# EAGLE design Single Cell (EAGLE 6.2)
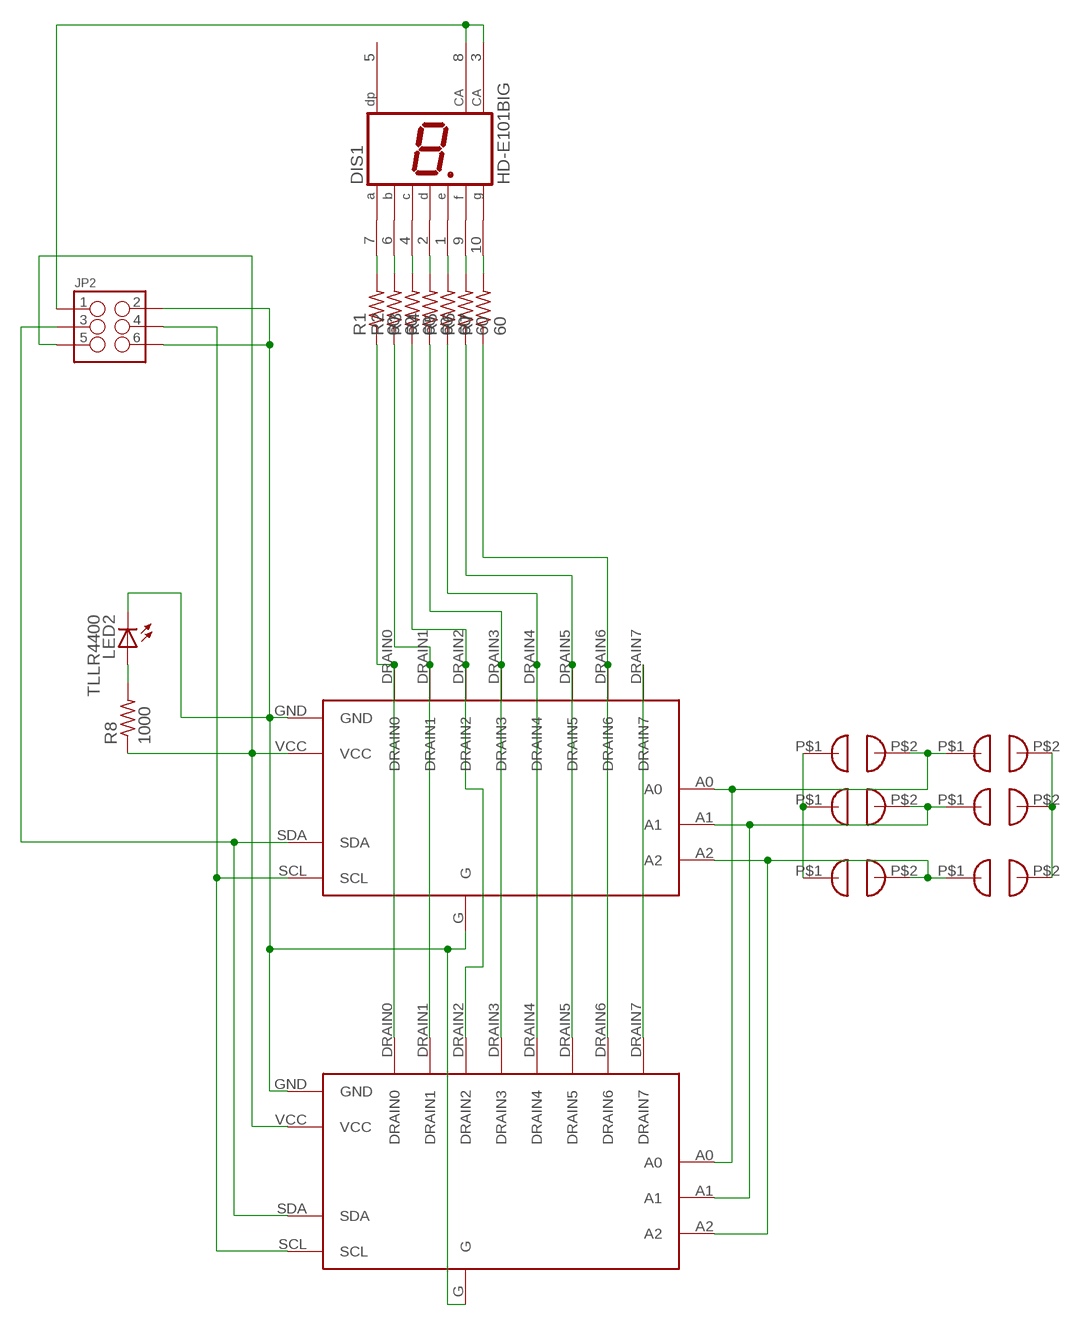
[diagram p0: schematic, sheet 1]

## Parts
DIS1  HD-E101BIG  HD-E101BACKWARDS  [7SEGMENT_BACKWARDS]
JP2  M03X2SHROUD  [2X3-SHROUDED]
LED2  TLLR4400  [LED3MM]
R1  60  R-US_0207/15  [0207/15]
R2  60  R-US_0207/15  [0207/15]
R3  60  R-US_0207/15  [0207/15]
R4  60  R-US_0207/15  [0207/15]
R5  60  R-US_0207/15  [0207/15]
R6  60  R-US_0207/15  [0207/15]
R7  60  R-US_0207/15  [0207/15]
R8  1000  R-US_0207/15  [0207/15]
U$1  SOLDER_JUMPER  [SOLDER_JUMPER]
U$2  LED_DRIVERBOARDADAFRUIT  [DRIVER_BOARD_ADAFRUIT]
U$3  SOLDER_JUMPER  [SOLDER_JUMPER]
U$4  SOLDER_JUMPER  [SOLDER_JUMPER]
U$5  SOLDER_JUMPER  [SOLDER_JUMPER]
U$6  SOLDER_JUMPER  [SOLDER_JUMPER]
U$7  SOLDER_JUMPER  [SOLDER_JUMPER]
U$8  LED_DRIVERBOARD  [DRIVER_BOARD]

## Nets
GND: JP2.2 JP2.6 LED2.K(C) U$1.P$1 U$2.G U$2.GND U$4.P$1 U$6.P$1 U$8.G U$8.GND
N$1: DIS1.7(A) R1.2
N$2: DIS1.6(B) R2.2
N$3: DIS1.4(C) R3.2
N$4: DIS1.2(D) R4.2
N$5: DIS1.1(E) R5.2
N$6: DIS1.9(F) R6.2
N$7: DIS1.10(G) R7.2
N$8: R1.1 U$2.DRAIN0 U$8.DRAIN0
N$9: R2.1 U$2.DRAIN1 U$8.DRAIN1
N$10: R3.1 U$2.DRAIN2 U$8.DRAIN2
N$11: R4.1 U$2.DRAIN3 U$8.DRAIN3
N$12: R5.1 U$2.DRAIN4 U$8.DRAIN4
N$13: R6.1 U$2.DRAIN5 U$8.DRAIN5
N$14: R7.1 U$2.DRAIN6 U$8.DRAIN6
N$15: U$2.A1 U$4.P$2 U$5.P$1 U$8.A1
N$16: U$2.A2 U$6.P$2 U$7.P$1 U$8.A2
N$17: U$2.DRAIN7 U$8.DRAIN7
N$18: LED2.A R8.2
N$29: U$1.P$2 U$2.A0 U$3.P$1 U$8.A0
SDA: JP2.3 U$2.SDA U$8.SDA
SSCL: JP2.4 U$2.SCL U$8.SCL
VCC5: JP2.5 R8.1 U$2.VCC U$3.P$2 U$5.P$2 U$7.P$2 U$8.VCC
VCC12: DIS1.3(CA) DIS1.8(CA) JP2.1
Unconnected: DIS1.5(DP)

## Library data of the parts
DIS1 = Parts:HD-E101: LED DISPLAY 1-character 7 segment, decimal point right
JP2 = Ben-SF-Con:M03X2: 2x3 .1" header. Shrouded, with keying- CONN-10681 SMT- CONN-11415 Pogo pins- HW-11044; PROD_ID: CONN-10681
LED2 = led:TLLR4400: Low Current (2mA) LED 3 mm Tinted Diffused Package color RED; MF: VISHAY SEMICONDUCTOR; OC_FARNELL: 1612437
R1-R8 = Ben-rcl:R-US_: RESISTOR, American symbol
U$1 U$3-U$7 = Parts:SOLDER_JUMPER
U$2 U$8 = Parts:LED_DRIVERBOARD

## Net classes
0 default: width 0.001 mm

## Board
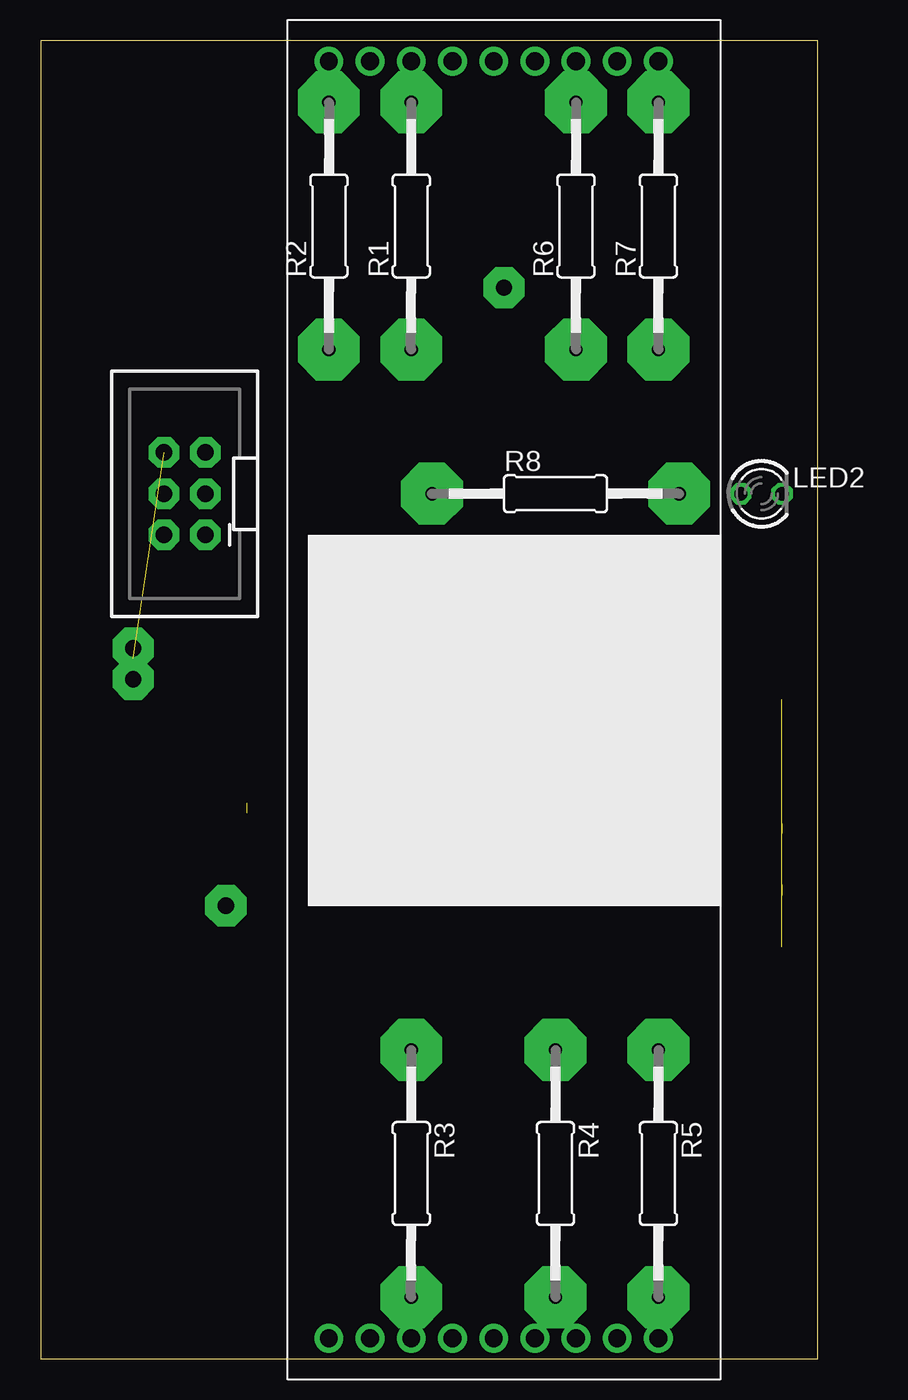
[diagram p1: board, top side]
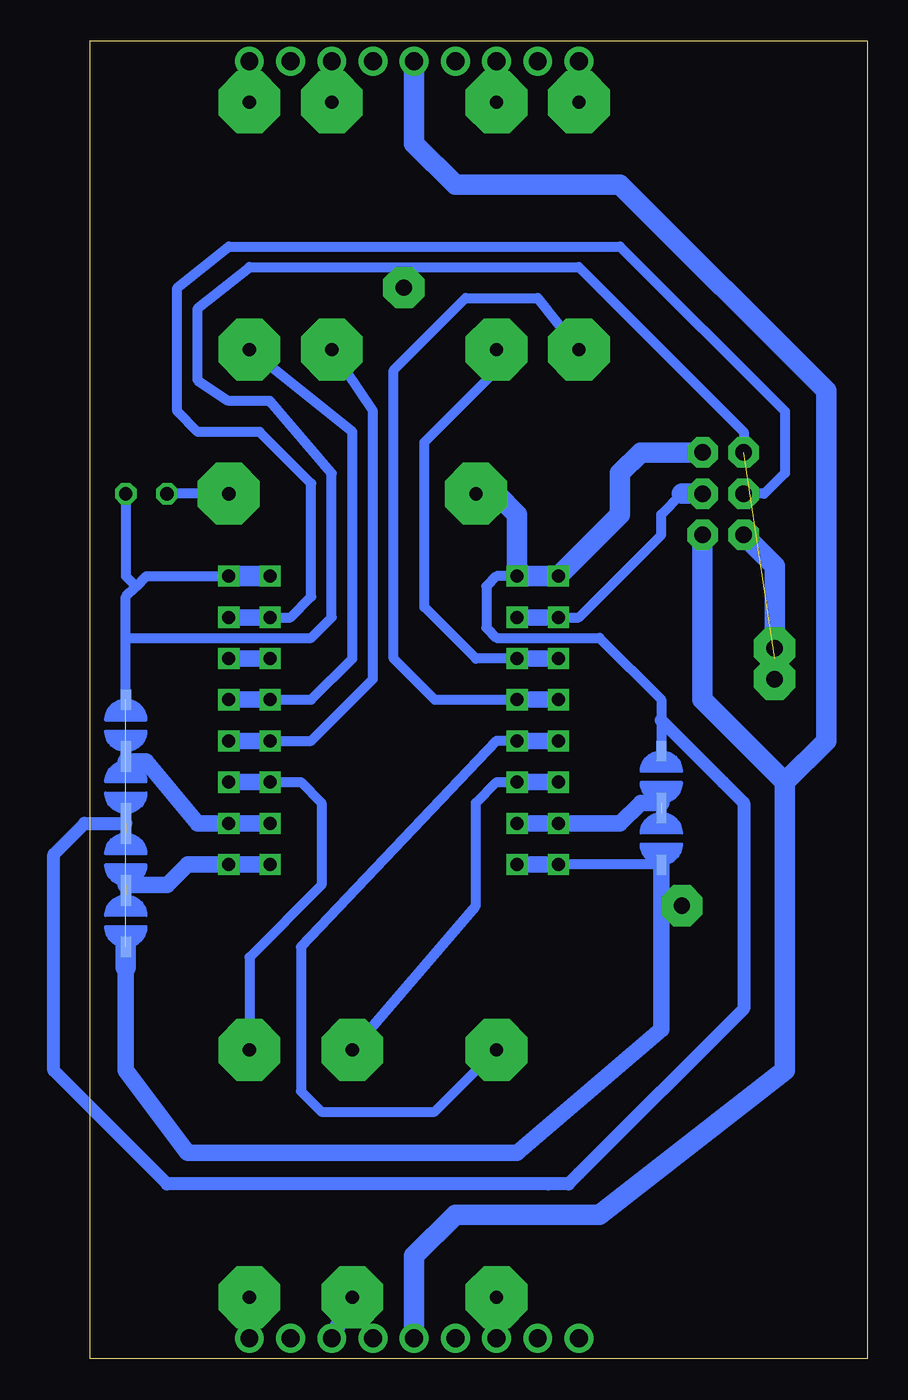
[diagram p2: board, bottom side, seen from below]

Size 47.93 x 81.27 mm. Coordinates in mm from the lower left corner, seen from the top.
Outline: 0,0 47.93,0 47.93,81.27 0,81.27 0,0
Copper layers (1*16): Top 0.035mm / dielectric 1.5mm / Bottom 0.035mm
Design rules: minimum track width 10mil, minimum drill 24mil, track to track 10mil, track to pad 10mil, pad to pad 10mil, via to via 10mil, smd to smd 10mil, copper to edge 40mil, drill to drill 8mil, minimum pad ring 10mil, minimum via ring 8mil, stop-mask expansion 4mil, vias tented up to drill 0mil, thermal gap 10mil

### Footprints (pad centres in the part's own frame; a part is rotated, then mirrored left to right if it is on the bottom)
7SEGMENT_BACKWARDS = drill 1.1 pad 1.778: 1 20.32,0; 2 15.24,0; 3 10.16,0; 4 5.08,0; 5 0,0; 6 0,78.74; 7 5.08,78.74; 8 10.16,78.74; 9 15.24,78.74; 10 20.32,78.74; GND 17.78,78.74; GND2 12.7,78.74; GND3 7.62,78.74; GND4 2.54,78.74; GND5 17.78,0; GND6 12.7,0; GND7 7.62,0; GND8 2.54,0
2X3-SHROUDED = drill 1.016 pad 1.88 octagon: 1 -1.27,2.54; 2 1.27,2.54; 3 -1.27,0; 4 1.27,0; 5 -1.27,-2.54; 6 1.27,-2.54
LED3MM = drill 0.813 octagon: A -1.27,0; K 1.27,0
0207/15 = drill 0.813 pad 3.81 octagon: 1 -7.62,0; 2 7.62,0
SOLDER_JUMPER = smd 0.635 x 1.27: P$1 0,1.27; P$2 0,-1.905
DRIVER_BOARD_ADAFRUIT = drill 0.8 square: A0 8.89,7.62; A1 6.35,7.62; A2 6.35,-7.62; DRAIN0 -3.81,-7.62; DRAIN1 -1.27,-7.62; DRAIN2 1.27,-7.62; DRAIN3 3.81,-7.62; DRAIN4 3.81,7.62; DRAIN5 1.27,7.62; DRAIN6 -1.27,7.62; DRAIN7 -3.81,7.62; G 8.89,-7.62; GND -8.89,7.62; SCL -6.35,7.62; SDA -6.35,-7.62; VCC -8.89,-7.62
DRIVER_BOARD = drill 0.8 square: A0 8.89,10.16; A1 6.35,10.16; A2 6.35,-10.16; DRAIN0 -3.81,-10.16; DRAIN1 -1.27,-10.16; DRAIN2 1.27,-10.16; DRAIN3 3.81,-10.16; DRAIN4 3.81,10.16; DRAIN5 1.27,10.16; DRAIN6 -1.27,10.16; DRAIN7 -3.81,10.16; G 8.89,-10.16; GND -8.89,10.16; SCL -6.35,10.16; SDA -6.35,-10.16; VCC -8.89,-10.16

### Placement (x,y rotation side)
DIS1  17.78,1.27 0 top
JP2  8.89,53.34 180 top
LED2  44.45,53.34 0 top
R1  22.86,69.85 90 top
R2  17.78,69.85 90 top
R3  22.86,11.43 270 top
R4  31.75,11.43 270 top
R5  38.1,11.43 270 top
R6  33.02,69.85 90 top
R7  38.1,69.85 90 top
R8  31.75,53.34 0 top
U$1  45.72,26.67 180 bottom
U$2  29.21,39.37 270 top
U$3  45.72,30.48 180 bottom
U$4  45.72,39.37 0 bottom
U$5  45.72,35.56 0 bottom
U$6  12.7,31.75 180 bottom
U$7  12.7,35.56 180 bottom
U$8  29.21,39.37 270 top

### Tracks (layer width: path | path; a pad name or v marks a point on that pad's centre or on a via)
GND  (3 unrouted)
  Bottom 0.61: U$6.P$1 | U$6.P$1 U$8.G | 45.72,44.45 45.72,46.99 | 45.72,46.99 45.09,47.63 | 45.09,47.63 44.45,48.26 U$8.GND | 45.72,46.99 | U$4.P$1 | U$4.P$1 45.72,44.45 | 45.72,44.45 34.29,44.45 33.02,45.72 33.02,54.61 36.83,59.06 39.37,59.06 41.28,60.33 41.28,64.77 38.1,67.31 17.78,67.31 7.62,57.15 JP2.6 | LED2.K | LED2.K 45.72,48.26 45.09,47.63
  Bottom 1.016: U$8.G U$2.G | 45.72,24.13 45.72,17.78 41.91,12.7 21.59,12.7 12.7,20.32 U$6.P$1 | U$1.P$1
  Bottom 1.27: U$2.GND U$8.GND | U$1.P$1 | U$1.P$1 45.72,24.13 | JP2.2 5.72,48.9 5.72,43.18
N$1
  Bottom 1.016: R1.2 DIS1.7
N$2
  Bottom 1.016: R2.2 DIS1.6
N$3
  Bottom 1.016: R3.2 DIS1.4
N$4
  Bottom 1.016: DIS1.2 | DIS1.2 R4.2
N$5
  Bottom 1.016: R5.2 DIS1.1 | DIS1.1
N$6
  Bottom 1.016: R6.2 DIS1.9 | DIS1.9
N$7
  Bottom 1.016: R7.2 DIS1.10 | DIS1.10
N$8
  Bottom 0.61: U$2.DRAIN0 | U$2.DRAIN0 24.13,43.18 27.31,46.35 27.31,56.51 22.86,60.96 R1.1
  Bottom 1.016: U$2.DRAIN0 U$8.DRAIN0
N$9
  Bottom 0.61: R2.1 20.32,65.41 24.77,65.41 29.21,60.96 29.21,43.18 26.67,40.64 U$2.DRAIN1 | U$2.DRAIN1
  Bottom 1.016: U$8.DRAIN1 U$2.DRAIN1
N$10
  Bottom 0.61: U$2.DRAIN2 | U$2.DRAIN2 22.86,38.1 34.93,25.4 34.93,16.51 33.66,15.24 26.67,15.24 R3.1
  Bottom 1.016: U$2.DRAIN2 U$8.DRAIN2
N$11
  Bottom 0.61: R4.1 24.13,27.94 24.13,34.29 22.86,35.56 U$2.DRAIN3
  Bottom 1.016: U$8.DRAIN3 U$2.DRAIN3
N$12
  Bottom 0.61: U$8.DRAIN4 | U$8.DRAIN4 34.93,35.56 33.66,34.29 33.66,29.21 38.1,24.77 R5.1
  Bottom 1.016: U$2.DRAIN4 | U$2.DRAIN4 U$8.DRAIN4 | U$8.DRAIN4 | U$8.DRAIN4
N$13
  Bottom 0.61: R6.1 30.48,58.42 30.48,41.91 31.75,40.64 34.29,38.1 | U$2.DRAIN5 34.29,38.1 | 34.29,38.1
  Bottom 1.016: U$8.DRAIN5 U$2.DRAIN5
N$14
  Bottom 0.61: U$2.DRAIN6 34.29,40.64 31.75,43.18 31.75,57.15 R7.1
  Bottom 1.016: U$2.DRAIN6 U$8.DRAIN6
N$15  (1 unrouted)
  Bottom 1.016: U$8.A1 | U$8.A1 41.28,33.02 44.45,36.83 U$5.P$1 | U$2.A1 U$8.A1
N$16  (1 unrouted)
  Bottom 1.016: U$7.P$1 13.97,34.29 15.24,33.02 U$8.A2 U$2.A2
N$17
  Bottom 1.016: U$8.DRAIN7 U$2.DRAIN7
N$18
  Bottom 0.61: R8.2 LED2.A
N$19  (via drill 1 pad 2.54)
  other vias: 5.72,41.91
N$20  (via drill 1 pad 2.54)
  other vias: 11.43,27.94
N$21  (via drill 1 pad 2.54)
  other vias: 5.72,43.81
N$22  (via drill 1 pad 2.54)
  other vias: 28.58,66.04
N$29  (1 unrouted)
  Bottom 1.016: 43.18,29.21 41.91,30.48 U$8.A0 U$2.A0 | 43.18,29.21 | 43.18,29.21 U$3.P$1
SDA
  Bottom 0.61: U$8.SDA 17.78,45.72 12.7,50.8 12.7,52.07 11.43,53.34
  Bottom 1.016: U$8.SDA U$2.SDA
  Bottom 1.27: 11.43,53.34 JP2.3
SSCL
  Bottom 0.61: U$2.SCL 35.56,45.72 34.29,46.99 34.29,53.98 37.47,57.15 40.64,57.15 41.28,57.15 42.55,58.42 42.55,66.04 39.37,68.58 15.24,68.58 5.08,58.42 5.08,54.61 6.35,53.34 JP2.4
  Bottom 1.016: U$2.SCL U$8.SCL
VCC5  (1 unrouted)
  Bottom 0.61: U$8.VCC | U$2.VCC 22.86,48.26 | 22.86,48.26 | 22.86,48.26 23.5,47.62 23.5,45.08 22.86,44.45 16.51,44.45 12.7,40.64 12.7,39.37 U$7.P$2 | U$5.P$2 45.72,33.02
  Bottom 0.813: 12.7,39.37 | 12.7,39.37 8.89,35.56 | 8.89,35.56 | 8.89,35.56 7.62,34.29 7.62,21.59 17.78,11.43 18.42,10.79 19.69,10.79 43.18,10.79 50.17,17.78 50.17,31.11 48.26,33.02 45.72,33.02
  Bottom 1.27: JP2.5 13.97,55.88 15.24,54.61 15.24,52.07 U$8.VCC U$2.VCC 21.59,52.07 22.86,53.34 R8.1
VCC12
  Bottom 1.27: JP2.1 | JP2.1 10.16,40.64 5.08,35.56 | 5.08,35.56 5.08,17.78 16.51,8.89 25.4,8.89 27.94,6.35 DIS1.3 | DIS1.8 27.94,74.93 25.4,72.39 15.24,72.39 2.54,59.69 2.54,38.1 5.08,35.56

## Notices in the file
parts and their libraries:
Ben-SF-Con: Licensing: CC v3.0 Share-Alike You are welcome to use this library for commercial purposes.
